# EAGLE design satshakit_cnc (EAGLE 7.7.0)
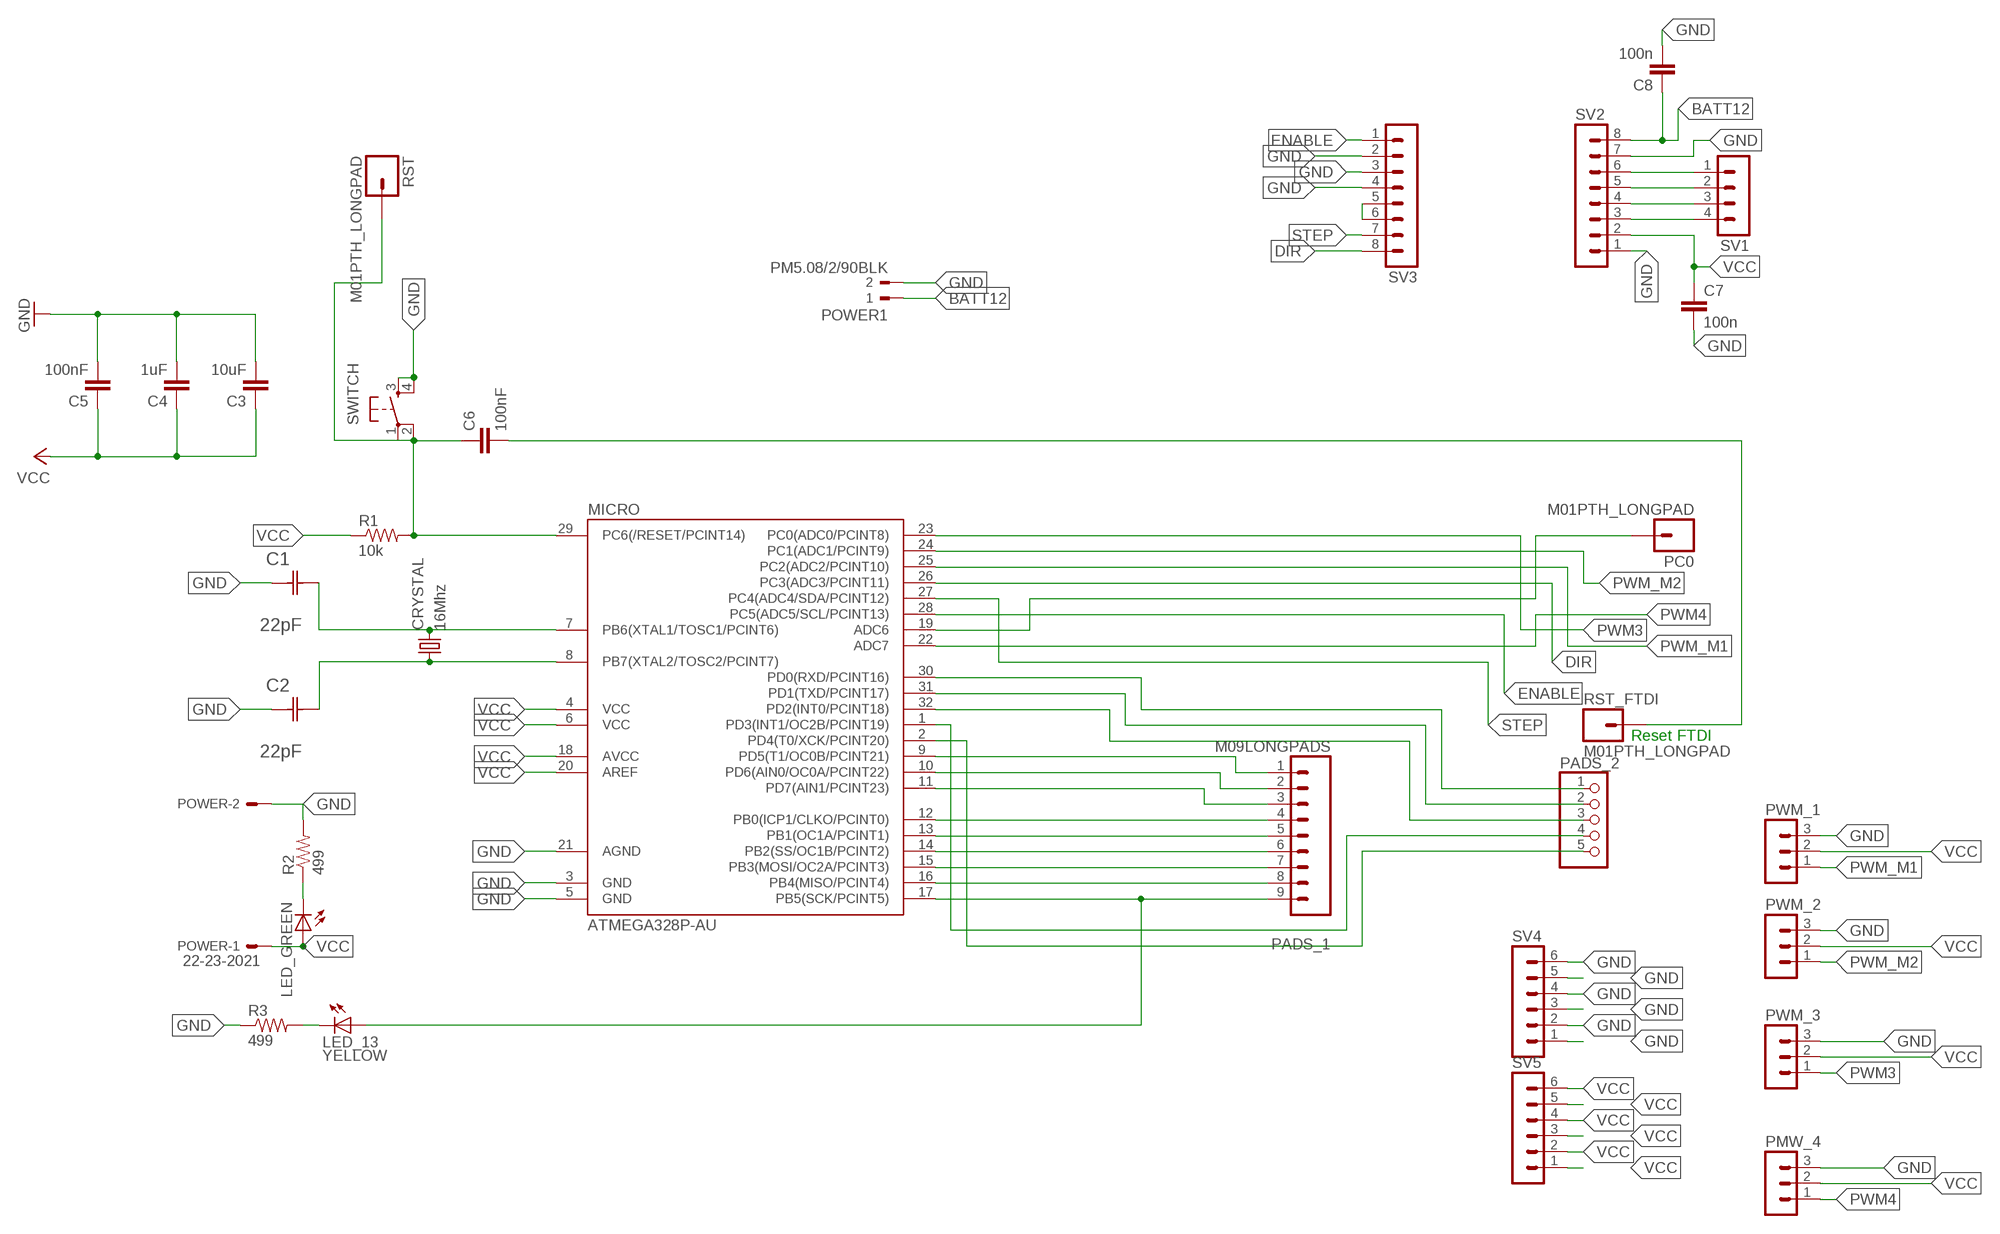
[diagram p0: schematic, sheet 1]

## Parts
C1  22pF  0612ZC225MAT2A  [CAPC3216X178N]
C2  22pF  0612ZC225MAT2A  [CAPC3216X178N]
C3  10uF  CAP1206  [1206]
C4  1uF  CAP1206  [1206]
C5  100nF  CAP1206  [1206]
C6  100nF  CAP1206  [1206]
C7  100n  CAP1206  [1206]
C8  100n  CAP1206  [1206]
CRYSTAL  16Mhz  CSM-7X-DU  [CSM-7X-DU]
LED_13  YELLOW  LED1206  [1206]
LED_GREEN  LED1206  [1206]
MICRO  ATMEGA328P-AU  ATMEGA48/88/168-AU  [TQFP32-08]
PADS_1  M09LONGPADS  [1X09_LONGPADS]
PADS_2  PINHD-1X5  [1X05]
PC0  M01PTH_LONGPAD  [1X01_LONGPAD]
PMW_4  MA03-1  [MA03-1]
POWER  22-23-2021  [22-23-2021]
POWER1  PM5.08/2/90BLK  [WEIDMULLER_PM5.08_2]
PWM_1  MA03-1  [MA03-1]
PWM_2  MA03-1  [MA03-1]
PWM_3  MA03-1  [MA03-1]
R1  10k  RESISTOR1206  [1206]
R2  499  RESISTOR1206  [1206]
R3  499  RESISTOR1206  [1206]
RST  M01PTH_LONGPAD  [1X01_LONGPAD]
RST_FTDI  M01PTH_LONGPAD  [1X01_LONGPAD]
SV1  MA04-1  [MA04-1]
SV2  MA08-1  [MA08-1]
SV3  MA08-1  [MA08-1]
SV4  MA06-1  [MA06-1]
SV5  MA06-1  [MA06-1]
SWITCH  6MM_SWITCH6MM_SWITCH  [6MM_SWITCH]

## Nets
BATT12: C8.1 POWER1.1 SV2.8
DIR: MICRO.26(PC3(ADC3/PCINT11)) SV3.8
ENABLE: MICRO.28(PC5(ADC5/SCL/PCINT13)) SV3.1
GND: C1.1(C1) C2.1(C1) C3.2 C4.2 C5.2 C7.2 C8.2 MICRO.3(GND) MICRO.5(GND) MICRO.21(AGND) PMW_4.3 POWER1.2 POWER.2 PWM_1.3 PWM_2.3 PWM_3.3 R2.2 R3.1 SV2.1 SV2.7 SV3.2 SV3.3 SV3.4 SV4.1 SV4.2 SV4.3 SV4.4 SV4.5 SV4.6 SWITCH.3(S) SWITCH.4(S1)
N$1: MICRO.9(PD5(T1/OC0B/PCINT21)) PADS_1.1
N$2: C1.2(C2) CRYSTAL.2 MICRO.7(PB6(XTAL1/TOSC1/PCINT6))
N$3: C6.2 RST_FTDI.1
N$4: MICRO.10(PD6(AIN0/OC0A/PCINT22)) PADS_1.2
N$5: MICRO.11(PD7(AIN1/PCINT23)) PADS_1.3
N$6: MICRO.12(PB0(ICP1/CLKO/PCINT0)) PADS_1.4
N$7: MICRO.13(PB1(OC1A/PCINT1)) PADS_1.5
N$8: MICRO.14(PB2(SS/OC1B/PCINT2)) PADS_1.6
N$9: C2.2(C2) CRYSTAL.1 MICRO.8(PB7(XTAL2/TOSC2/PCINT7))
N$10: MICRO.15(PB3(MOSI/OC2A/PCINT3)) PADS_1.7
N$11: MICRO.16(PB4(MISO/PCINT4)) PADS_1.8
N$12: LED_13.1(A) MICRO.17(PB5(SCK/PCINT5)) PADS_1.9
N$13: MICRO.19(ADC6) PC0.1
N$20: MICRO.30(PD0(RXD/PCINT16)) PADS_2.1
N$21: MICRO.31(PD1(TXD/PCINT17)) PADS_2.2
N$22: MICRO.32(PD2(INT0/PCINT18)) PADS_2.3
N$23: MICRO.1(PD3(INT1/OC2B/PCINT19)) PADS_2.4
N$24: MICRO.2(PD4(T0/XCK/PCINT20)) PADS_2.5
N$26: LED_GREEN.2(C) R2.1
N$27: LED_13.2(C) R3.2
N$28: C6.1 MICRO.29(PC6(/RESET/PCINT14)) R1.2 RST.1 SWITCH.1(P) SWITCH.2(P1)
N$35: SV3.5 SV3.6
N$38: SV1.1 SV2.6
N$39: SV1.2 SV2.5
N$40: SV1.3 SV2.4
N$41: SV1.4 SV2.3
PWM3: MICRO.23(PC0(ADC0/PCINT8)) PWM_3.1
PWM4: MICRO.22(ADC7) PMW_4.1
PWM_M1: MICRO.25(PC2(ADC2/PCINT10)) PWM_1.1
PWM_M2: MICRO.24(PC1(ADC1/PCINT9)) PWM_2.1
STEP: MICRO.27(PC4(ADC4/SDA/PCINT12)) SV3.7
VCC: C3.1 C4.1 C5.1 C7.1 LED_GREEN.1(A) MICRO.4(VCC) MICRO.6(VCC) MICRO.18(AVCC) MICRO.20(AREF) PMW_4.2 POWER.1 PWM_1.2 PWM_2.2 PWM_3.2 R1.1 SV2.2 SV5.1 SV5.2 SV5.3 SV5.4 SV5.5 SV5.6

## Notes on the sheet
- Reset FTDI

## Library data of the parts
C1 C2 = AVX_By_element14_Batch_1:0612ZC225MAT2A: Capacitor 1206; MPN: 0612ZC225MAT2A; OC_FARNELL: -; OC_NEWARK: 12N3209; SUPPLIER: AVX; TOLERANCE: ±20%; VALUE: 2.2µF; VOLTAGERATING: 10V
C3-C8 = 01_SparkFun:CAP: Capacitor
CRYSTAL = 01_FAB_Hello:CSM-7X-DU: SMD CRYSTAL; OC_FARNELL: unknown; OC_NEWARK: unknown
LED_13 LED_GREEN = 01_FAB_Hello:LED
MICRO = atmega8:ATMEGA48/88/168
PADS_1 = 01_SparkFun:M09: Header 9 Standard 9-pin 0.1" header. Use with straight break away headers (SKU : PRT-00116), right angle break away headers (PRT-00553), swiss pins (PRT-00743), machine pins (PRT-00117), and female headers (PRT-00115).
PADS_2 = pinhead:PINHD-1X5: PIN HEADER
PC0 RST RST_FTDI = 01_SparkFun:M01: Header 1
PMW_4 PWM_1-PWM_3 = con-lstb:MA03-1: PIN HEADER; OC_FARNELL: unknown; OC_NEWARK: unknown
POWER = con-molex:22-23-2021: .100" (2.54mm) Center Header - 2 Pin; MF: MOLEX; MPN: 22-23-2021; OC_FARNELL: 1462926; OC_NEWARK: 25C3832
POWER1 = WEIDMULLER-PM5.08_2_90BLK:PM5.08/2/90BLK: TERMINAL BLOCK, SIDE ENTRY, 2WAY; MPN: PM5.08/2/90 BLK; OC_FARNELL: 1131855; OC_NEWARK: 26M1980; PACKAGE: TH-R/A; SUPPLIER: WEIDMULLER
R1-R3 = 01_SparkFun:RESISTOR: Resistor
SV1 = con-lstb:MA04-1: PIN HEADER; OC_FARNELL: unknown; OC_NEWARK: unknown
SV2 SV3 = con-lstb:MA08-1: PIN HEADER; OC_FARNELL: unknown; OC_NEWARK: unknown
SV4 SV5 = con-lstb:MA06-1: PIN HEADER; OC_FARNELL: unknown; OC_NEWARK: unknown
SWITCH = 01_FAB_Hello:6MM_SWITCH: OMRON SWITCH

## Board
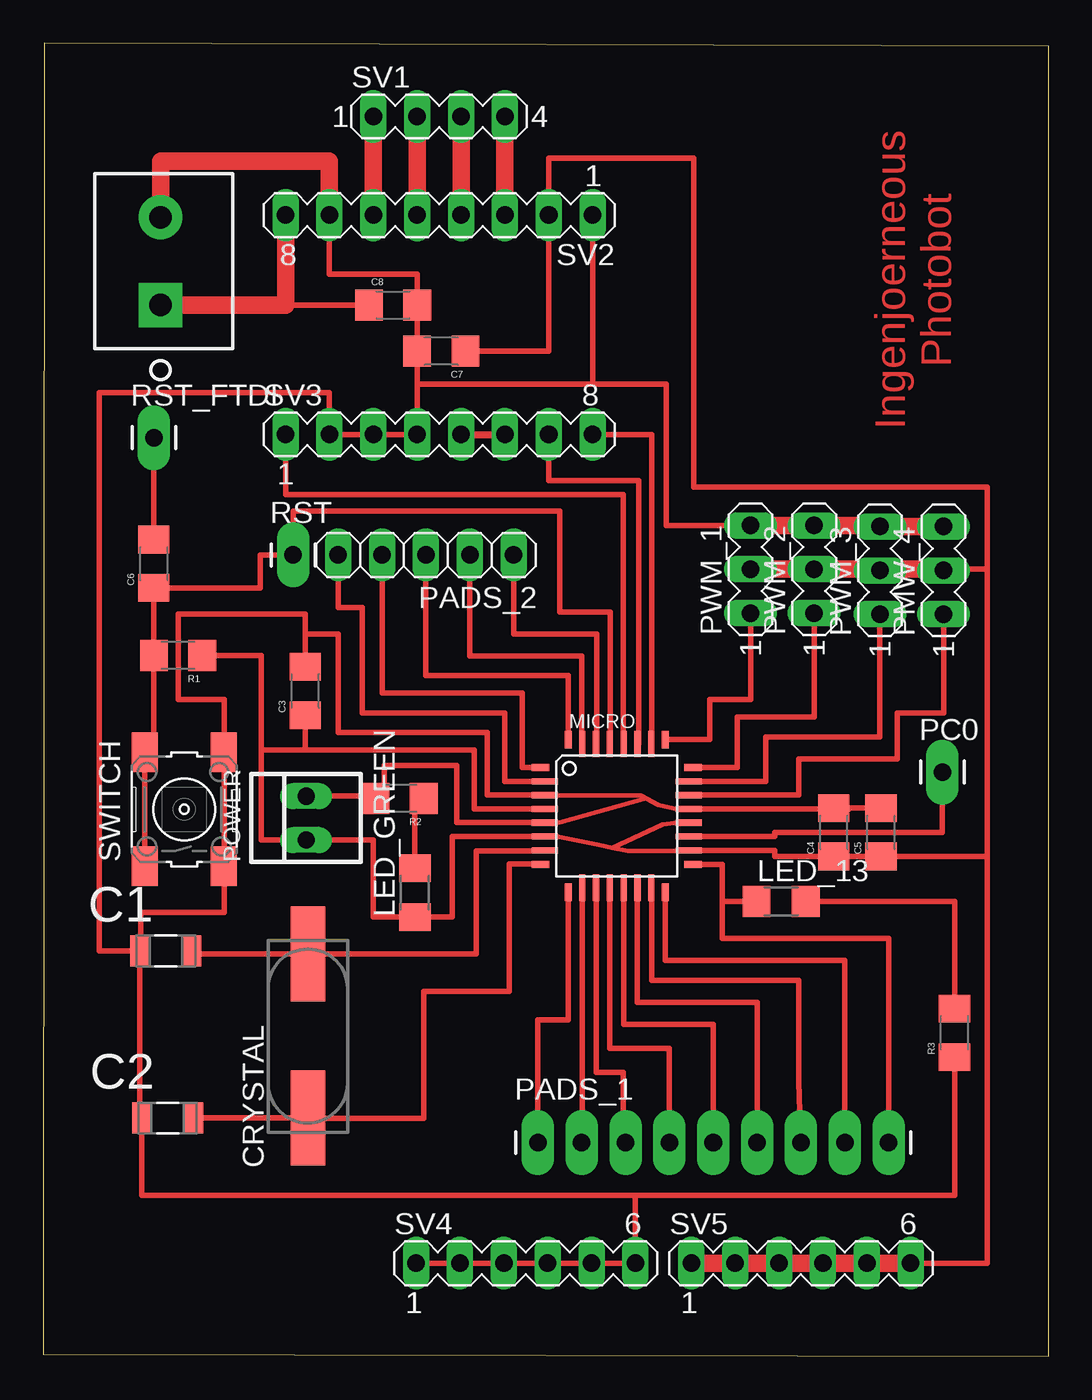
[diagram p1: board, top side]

Size 58.22 x 76.06 mm. Coordinates in mm from the lower left corner, seen from the top.
Outline: 0,0.13 58.22,0 58.22,75.87 0.06,76.06 0,0.13
Copper layers (1*16): Top 0.035mm / dielectric 1.5mm / Bottom 0.035mm
Design rules "default": minimum track width 10mil, minimum drill 24mil, track to track 8mil, track to pad 8mil, pad to pad 8mil, via to via 8mil, smd to smd 8mil, copper to edge 40mil, drill to drill 8mil, minimum pad ring 10mil, minimum via ring 8mil, stop-mask expansion 4mil, vias tented up to drill 0mil, thermal gap 10mil

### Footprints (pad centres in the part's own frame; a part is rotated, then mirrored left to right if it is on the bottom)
CAPC3216X178N = smd 1.118 x 1.803: 1 -1.499,0; 2 1.499,0
1206 = smd 1.6 x 1.8: 1 -1.4,0; 2 1.4,0
CSM-7X-DU = smd 5.5 x 2: 1 -4.75,0; 2 4.75,0
1206' = smd 1.6 x 1.803: 1 -1.422,0; 2 1.422,0
TQFP32-08 = smd 1.016 x 0.406: 1 -4.42,2.8; 8 -4.42,-2.8; 17 4.42,-2.8; 24 4.42,2.8 | smd 1.524 x 0.356: 2 -4.166,2; 3 -4.166,1.2; 4 -4.166,0.4; 5 -4.166,-0.4; 6 -4.166,-1.2; 7 -4.166,-2; 18 4.166,-2; 19 4.166,-1.2; 20 4.166,-0.4; 21 4.166,0.4; 22 4.166,1.2; 23 4.166,2 | smd 0.406 x 1.016: 9 -2.8,-4.42; 16 2.8,-4.42; 25 2.8,4.42; 32 -2.8,4.42 | smd 0.356 x 1.524: 10 -2,-4.166; 11 -1.2,-4.166; 12 -0.4,-4.166; 13 0.4,-4.166; 14 1.2,-4.166; 15 2,-4.166; 26 2,4.166; 27 1.2,4.166; 28 0.4,4.166; 29 -0.4,4.166; 30 -1.2,4.166; 31 -2,4.166
1X09_LONGPADS = drill 1.016 pad 1.88 long: 1 0,0; 2 2.54,0; 3 5.08,0; 4 7.62,0; 5 10.16,0; 6 12.7,0; 7 15.24,0; 8 17.78,0; 9 20.32,0
1X05 = drill 1.016 long: 1 -5.08,0; 2 -2.54,0; 3 0,0; 4 2.54,0; 5 5.08,0
1X01_LONGPAD = drill 1.016 pad 1.88 long: 1 0,0
MA03-1 = drill 1.016 long: 1 -2.54,0; 2 0,0; 3 2.54,0
22-23-2021 = drill 1 long: 1 -1.27,0; 2 1.27,0
WEIDMULLER_PM5.08_2 = drill 1.3 pad 2.54 square: 1 -2.54,0 | drill 1.3 pad 2.54: 2 2.54,0
MA04-1 = drill 1.016 long: 1 -3.81,0; 2 -1.27,0; 3 1.27,0; 4 3.81,0
MA08-1 = drill 1.016 long: 1 -8.89,0; 2 -6.35,0; 3 -3.81,0; 4 -1.27,0; 5 1.27,0; 6 3.81,0; 7 6.35,0; 8 8.89,0
MA06-1 = drill 1.016 long: 1 -6.35,0; 2 -3.81,0; 3 -1.27,0; 4 1.27,0; 5 3.81,0; 6 6.35,0
6MM_SWITCH = smd 2.286 x 1.524: 1 -3.302,2.286; 2 3.302,2.286; 3 -3.302,-2.286; 4 3.302,-2.286

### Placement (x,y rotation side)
C1  7.1,23.48 0 top
C2  7.2,13.8 0 top
C3  15.18,38.54 90 top
C4  45.78,30.35 90 top
C5  48.51,30.35 90 top
C6  6.41,45.91 90 top
C7  23.05,58.23 180 top
C8  20.26,60.9 0 top
CRYSTAL  15.33,18.55 90 top
LED_13  YELLOW  [1206']  42.74,26.35 0 top
LED_GREEN  [1206']  21.53,26.86 90 top
MICRO  33.21,31.31 0 top
PADS_1  28.64,12.38 0 top
PADS_2  22.16,46.42 180 top
PC0  52.07,33.85 0 top
PMW_4  52.13,45.53 90 top
POWER  15.23,31.18 90 top
POWER1  6.79,63.44 90 top
PWM_1  40.96,45.59 90 top
PWM_2  44.64,45.59 90 top
PWM_3  48.45,45.53 90 top
R1  7.81,40.6 180 top
R2  20.64,32.32 180 top
R3  52.77,18.73 90 top
RST  14.48,46.42 0 top
RST_FTDI  6.41,53.21 0 top
SV1  22.92,71.82 0 top
SV2  22.92,66.1 180 top
SV3  22.92,53.4 0 top
SV4  27.94,5.4 0 top
SV5  43.88,5.4 0 top
SWITCH  8.17,31.69 90 top

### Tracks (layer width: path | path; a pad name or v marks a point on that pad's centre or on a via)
BATT12
  Top 0.305: 14.03,60.9 C8.1
  Top 1.016: POWER1.1 14.03,60.9 SV2.8
DIR
  Top 0.305: SV3.8 35.24,53.4 35.24,35.47 MICRO.26 | SV3.8 31.75,53.4 31.75,53.47 31.81,53.47 SV3.8
ENABLE
  Top 0.305: SV3.1 14.03,49.91 33.59,49.91 33.59,35.47 MICRO.28
GND
  Top 0.254: MICRO.3 29.07,32.48 34.6,32.48 | 34.6,32.48 35.62,31.94 36.77,31.69 | 29.65,30.92 29.91,30.92 34.78,32.27 | 34.78,32.27 34.92,32.31 | 34.6,32.48 34.78,32.27
  Top 0.305: MICRO.5 | MICRO.21 | C1.1 5.6,13.8 C2.1 5.7,9.34 34.29,9.34 | C1.1 5.53,23.48 | MICRO.5 29.05,30.92 23.94,30.92 23.94,34.23 19.75,34.23 19.75,32.19 R2.2 19.75,32.45 POWER.2 | C1.1 5.65,23.48 5.65,25.72 10.48,25.72 10.48,28.38 | MICRO.21 46.67,31.71 C4.2 C5.2 | 29.65,30.92 MICRO.5 | MICRO.21 36.77,31.69 | MICRO.3 25.72,32.51 25.72,36.13 17.08,36.13 17.08,41.85 15.18,41.85 | C3.2 15.18,41.85 | 34.29,9.34 52.77,9.34 R3.1 | SWITCH.3 10.48,28.38 | 10.48,28.38 10.48,34.35 10.45,34.35 SWITCH.4 10.48,34.99 10.48,38.04 7.81,38.04 7.81,42.99 15.18,42.99 15.18,41.85 | C1.1 3.24,23.48 3.24,55.82 16.57,55.82 SV3.2 SV3.3 SV3.4 | 21.65,56.32 C7.2 C8.2 | 21.65,56.32 SV3.4 | 21.65,60.77 21.65,62.67 16.57,62.67 SV2.7 | SV4.1 SV4.2 SV4.3 SV4.4 SV4.5 SV4.6 34.29,9.34 | 21.65,56.32 31.81,56.32 | 31.81,56.32 36.07,56.32 36.07,48.13 PWM_1.3 | SV2.1 31.81,56.32
  Top 0.406: SV3.4 | C8.2 21.65,60.77
  Top 1.016: PWM_1.3 PWM_2.3 48.45,48.13 PWM_3.3 PMW_4.3 | POWER1.2 6.79,69.22 16.57,69.22 SV2.7
N$1
  Top 0.305: PADS_1.1 28.64,19.49 30.41,19.49 MICRO.9
N$2
  Top 0.305: 8.6,23.3 C1.2 8.6,23.3 | MICRO.7 29.05,29.27 25.08,29.27 25.08,23.3 CRYSTAL.2 8.6,23.3
N$3
  Top 0.305: C6.2 RST_FTDI.1
N$4
  Top 0.305: PADS_1.2 31.21,15.94 MICRO.10
N$5
  Top 0.305: MICRO.11 32.01,16.45 33.59,16.45 33.59,13.02 33.72,13.02 PADS_1.3
N$6
  Top 0.305: 32.83,27.14 MICRO.12 32.81,17.84 36.26,17.84 PADS_1.4
N$7
  Top 0.305: PADS_1.5 38.8,19.24 33.61,19.24 MICRO.13
N$8
  Top 0.305: PADS_1.6 41.34,20.51 34.41,20.51 MICRO.14
N$9
  Top 0.305: 8.7,13.78 C2.2 | MICRO.8 26.99,28.51 26.99,21.14 22.03,21.14 22.03,13.78 15.33,13.78 CRYSTAL.1 C2.2 | C2.2
N$10
  Top 0.305: PADS_1.7 43.75,15.94 43.75,21.78 35.24,21.78 35.24,26.35 MICRO.15
N$11
  Top 0.305: MICRO.16 36.01,22.92 46.42,22.92 PADS_1.8
N$12
  Top 0.305: PADS_1.9 48.96,24.19 39.31,24.19 39.31,26.35 | LED_13.1 39.31,26.35 | MICRO.17 39.31,28.5 39.31,26.35
N$13
  Top 0.305: MICRO.19 42.35,30.1 42.35,30.35 52.07,30.35 PC0.1
N$20
  Top 0.305: MICRO.30 32.07,35.47 32.07,41.85 27.24,41.85 PADS_2.1
N$21
  Top 0.305: MICRO.31 31.18,35.47 31.18,40.58 24.7,40.58 PADS_2.2
N$22
  Top 0.305: MICRO.32 30.42,39.43 22.16,39.43 PADS_2.3
N$23
  Top 0.305: MICRO.1 27.75,34.11 27.75,38.42 19.62,38.42 PADS_2.4
N$24
  Top 0.305: MICRO.2 26.73,33.3 26.73,37.28 18.48,37.28 18.48,43.37 17.08,43.37 PADS_2.5
N$26
  Top 0.305: 22.41,32.07 R2.1 22.04,31.94 21.53,31.94 LED_GREEN.2
N$27
  Top 0.305: LED_13.2 52.77,26.35 R3.2
N$28
  Top 0.305: MICRO.29 32.83,35.47 32.83,43.12 29.91,43.12 29.91,48.71 29.91,48.96 14.48,48.96 RST.1 12.57,46.42 12.57,44.51 C6.1 R1.2 | R1.2 6.16,40.6 | R1.2 6.41,34.99 SWITCH.2 SWITCH.1
N$35
  Top 0.406: SV3.5 SV3.6
N$38
  Top 1.016: SV2.6 SV1.1
N$39
  Top 1.016: SV2.5 SV1.2
N$40
  Top 1.016: SV1.3 SV2.4
N$41
  Top 1.016: SV2.3 SV1.4
PWM3
  Top 0.305: MICRO.23 41.85,33.3 41.85,35.88 48.45,35.88 PWM_3.1
PWM4
  Top 0.305: MICRO.22 43.75,32.51 43.75,34.61 49.47,34.61 49.47,37.28 52.13,37.28 PMW_4.1
PWM_M1
  Top 0.305: MICRO.25 38.61,35.73 38.61,38.04 40.96,38.04 PWM_1.1
PWM_M2
  Top 0.305: MICRO.24 40.2,34.11 40.2,37.02 44.64,37.02 PWM_2.1
STEP
  Top 0.305: MICRO.27 34.48,35.47 34.48,50.74 29.27,50.74 SV3.7
VCC
  Top 0.254: 29.73,30.11 32.19,29.61 32.94,29.46 | 32.94,29.46 33.84,29.27 37.38,29.27 | MICRO.20 36.77,30.91 36.77,30.92 35.88,30.8 32.94,29.46
  Top 0.305: MICRO.18 | MICRO.20 36.77,30.92 | MICRO.4 24.95,31.71 24.95,35.12 15.18,35.12 | 12.64,35.12 12.64,40.6 R1.1 | 12.64,35.12 12.64,29.91 POWER.1 19.11,29.91 19.11,25.44 LED_GREEN.1 21.53,25.46 23.69,25.46 23.69,30.11 MICRO.6 29.73,30.11 | 37.38,29.27 MICRO.18 | MICRO.18 42.35,29.3 42.35,28.95 C4.1 C5.1 | 12.64,35.12 15.18,35.12 | 15.18,35.12 C3.1 15.56,37.14 15.56,36.89 | C7.1 29.27,58.23 SV2.2 | SV2.2 29.27,69.34 | SV2.2 29.27,69.41 37.66,69.41 37.66,50.36 54.67,50.36 54.67,45.66 54.67,45.59 | SV5.5 54.67,5.4 54.67,28.96 | 54.67,28.96 C5.1 | PWM_1.2 54.67,45.59 | 54.67,28.96 54.67,45.53 54.67,45.59
  Top 1.016: PWM_1.2 PWM_2.2 48.45,45.59 | 48.45,45.59 PWM_3.2 | 48.45,45.59 52.13,45.59 PMW_4.2 | C5.1 | SV5.1 SV5.2 SV5.3 SV5.4 SV5.5 SV5.6

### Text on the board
Top: Ingenjoerneous / Photobot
